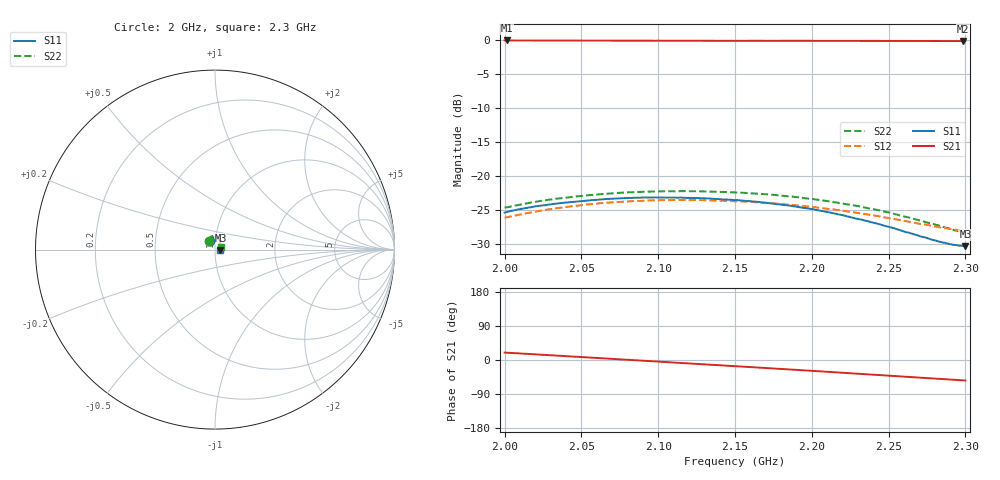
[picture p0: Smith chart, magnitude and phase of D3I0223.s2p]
! 11/4/2020 10:24:47 AM
! C:\USERS\DITOM\DESKTOP\SINGLE JUNCTION ISOLATOR DATA\2.0-2.3 GHZ (D3I0223).S2P
! CHANNEL.1
! TR.MEASUREMENT
! CORRECTED.DATA
# GHZ S RI R 50.0
! FREQ.GHZ  S11RE  S11IM  S21RE  S21IM  S12RE  S12IM  S22RE  S22IM
!; PortSelection: Port_12
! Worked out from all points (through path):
!   601 points, 2 GHz to 2.3 GHz, reference 50 ohm
!   highest |S21| = -0.13 dB at 2.002 GHz (marker M1); lowest = -0.2 dB at 2.299 GHz (marker M2)
!   lowest |S11| = -30.3 dB at 2.3 GHz (marker M3), VSWR 1.06, Z = 53.2 - j0.299 ohm
!   |S11| at or under -10 dB: start of sweep to end of sweep
!   |S22| runs from -28.3 to -22.2 dB; largest |S21 - S12| = 0.99
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2  -0.0251 0.0479  0.9279 0.33  -0.0059 0.0492  -0.0338 0.0482
2.0015  -0.0251 0.0486  0.9296 0.3255  -0.00589 0.0497  -0.0337 0.0485
2.0095  -0.0242 0.0518  0.9395 0.2941  -0.00516 0.052  -0.0332 0.0519
2.021  -0.0231 0.0557  0.9517 0.2485  -0.00353 0.0551  -0.0322 0.0566
2.033  -0.0211 0.0591  0.963 0.2009  -0.00157 0.058  -0.0306 0.0609
2.0505  -0.0175 0.0635  0.9739 0.1311  0.00207 0.0613  -0.0271 0.0665
2.073  -0.0127 0.0675  0.9812 0.0389  0.0076 0.0641  -0.0218 0.072
2.0905  -0.0079 0.0693  0.9809 -0.0336  0.0122 0.065  -0.0169 0.075
2.1  -0.00524 0.0696  0.9789 -0.0721  0.0146 0.0651  -0.0142 0.076
2.1315  0.00379 0.0686  0.9589 -0.2002  0.0221 0.0628  -0.00382 0.0771
2.15  0.00917 0.0661  0.9399 -0.2744  0.0257 0.0603  0.00243 0.0758
2.164  0.0134 0.0635  0.9222 -0.3297  0.0279 0.058  0.00733 0.0742
2.175  0.0168 0.0607  0.9058 -0.3724  0.0293 0.056  0.0109 0.0721
2.2  0.0231 0.0525  0.8602 -0.4684  0.0312 0.0507  0.0189 0.0653
2.2195  0.0273 0.0441  0.8157 -0.5393  0.0314 0.0464  0.0245 0.0582
2.229  0.0287 0.0395  0.7922 -0.5728  0.0309 0.0442  0.027 0.0542
2.236  0.0299 0.0362  0.7744 -0.5968  0.0305 0.0427  0.0286 0.051
2.25  0.0314 0.0287  0.7354 -0.6434  0.0289 0.04  0.0316 0.044
2.2825  0.032 0.00884  0.6323 -0.7432  0.0228 0.0357  0.0355 0.0252
2.2915  0.0314 0.00287  0.6015 -0.7679  0.0207 0.0353  0.0356 0.0194
2.2985  0.0308 -0.00169  0.5766 -0.7858  0.019 0.0349  0.0358 0.0147
2.3  0.0306 -0.00281  0.5712 -0.7898  0.0186 0.0349  0.0357 0.0139
